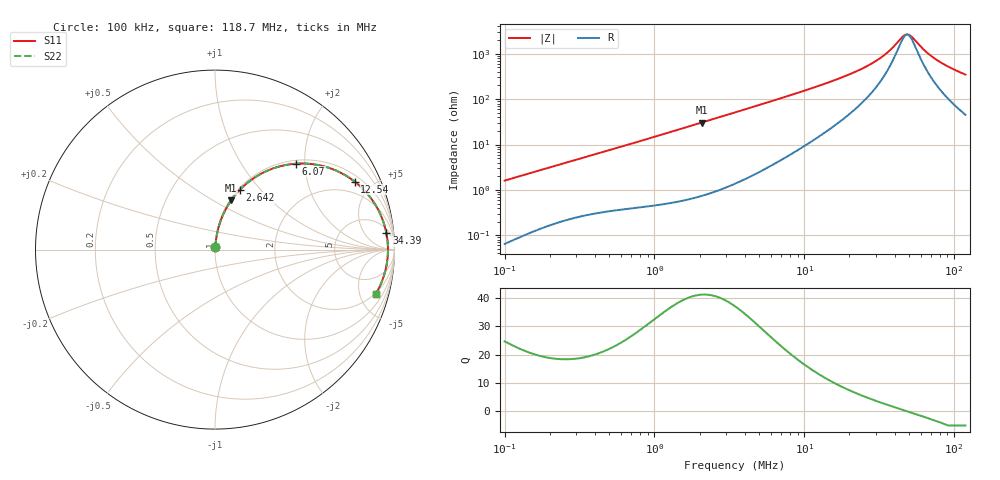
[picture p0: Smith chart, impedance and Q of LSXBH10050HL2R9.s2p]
! LSXBH10050HL2R9  S-PARAMETER MODEL  ( General Type )
! Model Generated by TAIYO YUDEN Corporation (http://www.ty-top.com)
! Version 3.0
! TAIYO YUDEN Control No. 180118NI43SB-FBB
! Copyright(c) 2007 TAIYO YUDEN CO.,LTD. All Rights Reserved.
! Product Description (link to TY-COMPAS)
! https://ds.yuden.co.jp/TYCOMPAS/or/detail?pn=LSXBH10050HL2R9N&u=M
! Products Name : Inductors
! Characteristics :
!  Inductance : 2.9 uH , SRF(min) : 29 MHz , DC Resistance(max) : 0.01209 Ohm
!  Rated Current : Saturation :8200 mA , Temp Rise : 7300 mA (40 degC)
!  Case Size : 10.0 x 9.8 / 0.394 x 0.386 [mm/inch] , Thickness : 5 / 0.197 [mm/inch]
!  (Conditions: Temperature = 25 degC , DC Bias Current/Voltage = 0A / 0V)
! External Node Assignments :
!  1  o---GGG---o  2
! GND o---------o GND
! Frequency Range : 0.1MHz  -  118.695536MHz  [ 402 STEP ]
# MHz S RI R 50
! Freq[MHz].  S11 Real  S11 Imag  S21 Real  S21 Imag  S12 Real  S12 Imag  S22 Real  S22 Imag
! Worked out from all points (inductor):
!   401 points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, 100 kHz to 118.7 MHz, reference 50 ohm
!   read as one part in series: L = 2.54 uH near 103.6 kHz
!   highest Q = 41.2 at 2.062 MHz (marker M1), where L = 2.35 uH
!   self-resonance near 48.52 MHz
!   S11 on the Smith chart (normalised r, x): 100 kHz: 1.00, +0.03; 2.642 MHz: 1.02, +0.78; 6.07 MHz: 1.07, +1.81; 12.54 MHz: 1.30, +3.93; 34.39 MHz: 8, +18; 118.7 MHz: 1.91, -6.88
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0.1  0.000905 0.016  0.9991 -0.016  0.9991 -0.016  0.000905 0.016
0.327316  0.00511 0.0496  0.9949 -0.0496  0.9949 -0.0496  0.00511 0.0496
1.07136  0.0288 0.1532  0.9712 -0.1532  0.9712 -0.1532  0.0288 0.1532
2.062152  0.0903 0.2747  0.9097 -0.2747  0.9097 -0.2747  0.0903 0.2747
2.641958  0.1381 0.3329  0.8619 -0.3329  0.8619 -0.3329  0.1381 0.3329
3.445222  0.2123 0.3957  0.7877 -0.3957  0.7877 -0.3957  0.2123 0.3957
6.069766  0.4529 0.4789  0.5471 -0.4789  0.5471 -0.4789  0.4529 0.4789
8.200407  0.6011 0.4653  0.3989 -0.4653  0.3989 -0.4653  0.6011 0.4653
11.27678  0.7396 0.4059  0.2604 -0.4059  0.2604 -0.4059  0.7396 0.4059
12.54011  0.7781 0.379  0.2219 -0.379  0.2219 -0.379  0.7781 0.379
22.88908  0.918 0.2042  0.082 -0.2042  0.082 -0.2042  0.918 0.2042
28.81028  0.9431 0.1388  0.0569 -0.1388  0.0569 -0.1388  0.9431 0.1388
34.38811  0.955 0.0905  0.045 -0.0905  0.045 -0.0905  0.955 0.0905
36.91074  0.9583 0.0716  0.0417 -0.0716  0.0417 -0.0716  0.9583 0.0716
45.64422  0.9634 0.0159  0.0366 -0.0159  0.0366 -0.0159  0.9634 0.0159
48.13312  0.9637 0.00205  0.0363 -0.00205  0.0363 -0.00205  0.9637 0.00205
49.86734  0.9637 -0.00716  0.0363 0.00716  0.0363 0.00716  0.9637 -0.00716
52.58652  0.9633 -0.021  0.0367 0.021  0.0367 0.021  0.9633 -0.021
63.88831  0.9583 -0.0722  0.0417 0.0722  0.0417 0.0722  0.9583 -0.0722
73.60547  0.951 -0.1102  0.049 0.1102  0.049 0.1102  0.951 -0.1102
92.64654  0.9312 -0.1743  0.0688 0.1743  0.0688 0.1743  0.9312 -0.1743
118.6955  0.8959 -0.2466  0.1041 0.2466  0.1041 0.2466  0.8959 -0.2466
